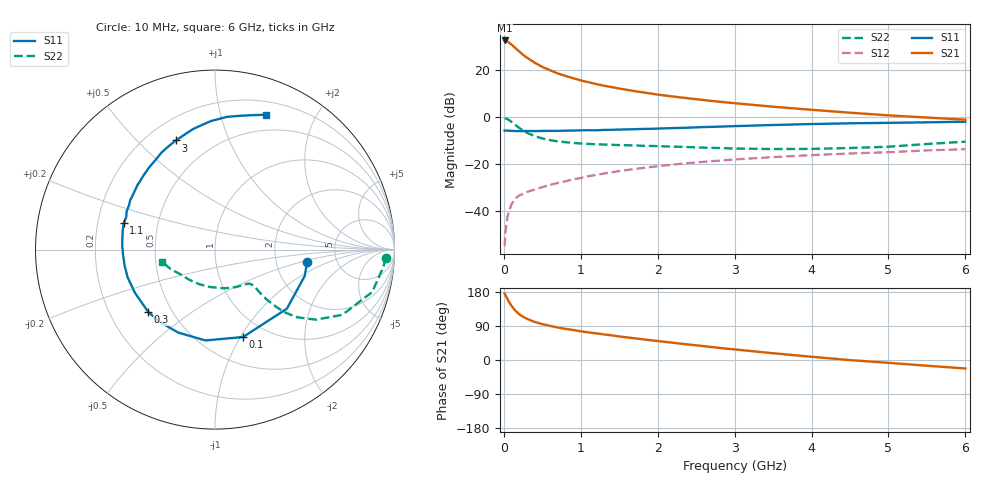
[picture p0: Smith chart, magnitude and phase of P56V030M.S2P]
! SIEMENS Small Signal Semiconductors
! BFP183
! Si NPN RF Bipolar Junction Transistor in SOT143
! VCE = 6 V  IC = 30 mA
! Common Emitter S-Parameters:  March  1996
# GHz  S  MA  R  50
!  f  S11  S21  S12  S22
! GHz  MAG  ANG  MAG  ANG  MAG  ANG  MAG  ANG
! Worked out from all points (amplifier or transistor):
!   36 points, 10 MHz to 6 GHz, reference 50 ohm
!   highest |S21| = 32.7 dB at 10 MHz (marker M1)
!   |S21| within 3 dB of that: start of sweep to 142.4 MHz
!   unconditionally stable (mu >= 1): 714.1 MHz to 5.748 GHz
!   at 250 MHz: K = 0.55, MSG = 29.6 dB, |S12| = -32.7 dB
!   at 1.4 GHz: K = 1.14, MAG = 15.9 dB, |S12| = -23.5 dB
!   at 6 GHz: K = 0.97, MSG = 6.3 dB, |S12| = -13.6 dB
!   S11 on the Smith chart (normalised r, x): 10 MHz: 3.04, -0.56; 100 MHz: 0.78, -1.03; 300 MHz: 0.37, -0.35; 1.1 GHz: 0.31, +0.13; 3 GHz: 0.31, +0.66; 6 GHz: 0.33, +1.39
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0.01  0.5185 -7.5  43.05 175.4  0.0018 80.9  0.9523 -2.8
0.02  0.5209 -16.4  42.89 171.6  0.0035 80.5  0.9425 -6.0
0.05  0.5185 -39.4  40.85 159.5  0.0081 78.3  0.9072 -15.1
0.1  0.5114 -72.2  35.16 142.8  0.0142 63.7  0.7973 -27.1
0.15  0.5089 -96.0  29.71 130.1  0.0185 57.3  0.6841 -34.8
0.2  0.5058 -113.9  25.09 120.9  0.0217 53.8  0.5927 -39.5
0.25  0.5068 -127.2  21.34 113.9  0.0233 51.3  0.5222 -42.0
0.3  0.509 -137.0  18.53 108.8  0.0257 51.3  0.4669 -43.1
0.4  0.507 -151.6  14.51 100.6  0.0289 51.3  0.3966 -44.0
0.5  0.5108 -162.4  11.78 94.7  0.0325 51.9  0.3537 -43.9
0.6  0.5114 -169.9  10 89.9  0.0361 53.3  0.325 -43.5
0.7  0.5131 -176.9  8.567 85.8  0.0397 54.3  0.3062 -43.2
0.8  0.5172 177.6  7.58 82.2  0.0432 55.1  0.294 -43.2
1  0.5254 167.9  6.081 75.8  0.0508 56.2  0.276 -44.1
1.1  0.5292 163.6  5.558 72.8  0.0555 55.6  0.2699 -44.7
1.5  0.5468 149.8  4.078 62.1  0.0716 54.8  0.2552 -49.3
2.2  0.5866 128.9  2.757 45.4  0.0981 49.8  0.2362 -62.4
3  0.6461 109.7  1.987 27.9  0.1261 42.4  0.2155 -82.8
3.5  0.683 100.3  1.673 17.8  0.1415 37.8  0.2101 -97.9
4.5  0.7424 84.9  1.248 -0.3  0.1686 28.4  0.2212 -130.8
5.5  0.7786 74.2  0.984 -15.1  0.1967 20.6  0.2693 -156.0
6  0.803 69.3  0.887 -22.4  0.2086 15.9  0.3016 -166.7
